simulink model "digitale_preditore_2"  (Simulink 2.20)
settings: Solver=VariableStepDiscrete  StartTime=0.0  StopTime=10.0  RelTol=1e-3  AbsTol=1e-6
libraries: Puma x1

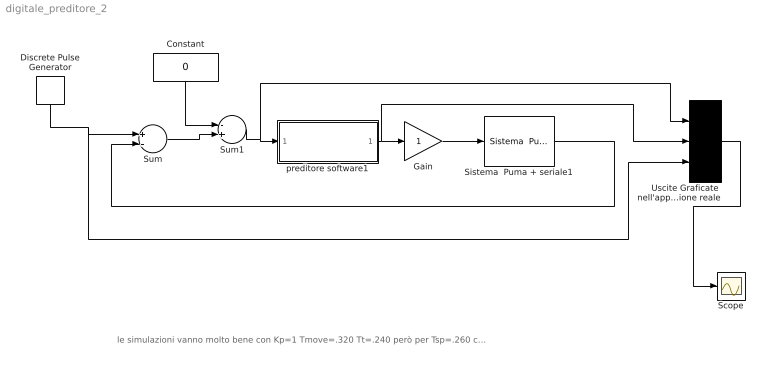
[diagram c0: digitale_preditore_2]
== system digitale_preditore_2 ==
  note: le simulazioni vanno molto bene con Kp=1 Tmove=.320 Tt=.240 però per Tsp=.260 c'è un punto ad alta sensibilità
  Constant : Constant  Orientation=down  Value=0
  Discrete Pulse Generator : DiscretePulseGenerator  Orientation=down  Amplitude=48  Period=100  PulseWidth=100  PhaseDelay=1  SampleTime=.1
  Gain : Gain  Gain=1
  Scope : Scope
  Sistema  Puma + seriale1 : Puma/Sistema  Puma + seriale  Ts=.260
  Sum : Sum  Inputs=+-
  Sum1 : Sum  Inputs=-+
  Uscite Graficate  nell'applicazione reale : Mux  Inputs=3
  preditore software1 : Subsystem  mask(Modello dinamico preditivo del Puma 260 + ritardo seriale){Tsp=.260, Tt=.330}
      mask prompts: Tsp "Sample Time Tsp del preditore"; Tt "Ritardo Totale Tt del sistema da modellare"
      mask help: Preditore della posizione del Puma all'istante successivo. Questo viene effettuato tramite la conoscenza 1) dell'ingresso all'istante precedente 2) della posizione presente del Puma (ottenuta dalla ripresa dalla telecamera).
      mask init:
      | if exist('Tt')== 0
      | Tt=.320;
      | end
      | if exist('Tsp')== 0
      | Tsp=.260;
      | end
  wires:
  Sum/1 -> Sum1/2
  Constant/1 -> Sum1/1
  Sum1/1 -> Uscite Graficate  nell'applicazione reale/1, preditore software1/1(In1)
  preditore software1/1(Out1) -> Gain/1, Uscite Graficate  nell'applicazione reale/2
  Discrete Pulse Generator/1 -> Sum/1, Uscite Graficate  nell'applicazione reale/3
  Uscite Graficate  nell'applicazione reale/1 -> Scope/1
  Sistema  Puma + seriale1/1 -> Sum/2
  Gain/1 -> Sistema  Puma + seriale1/1

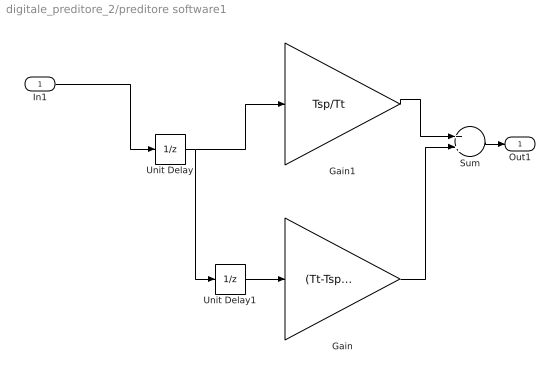
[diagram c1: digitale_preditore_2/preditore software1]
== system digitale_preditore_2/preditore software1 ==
  In1 : Inport  Port=1  PortWidth=-1  SampleTime=-1
  Gain : Gain  Gain=(Tt-Tsp)/Tt
  Gain1 : Gain  Gain=Tsp/Tt
  Sum : Sum  Inputs=++
  Unit Delay : UnitDelay  X0=0  SampleTime=Tsp
  Unit Delay1 : UnitDelay  X0=0  SampleTime=Tsp
  Out1 : Outport  Port=1
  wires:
  Sum/1 -> Out1/1
  In1/1 -> Unit Delay/1
  Unit Delay1/1 -> Gain/1
  Gain1/1 -> Sum/1
  Gain/1 -> Sum/2
  Unit Delay/1 -> Gain1/1, Unit Delay1/1
